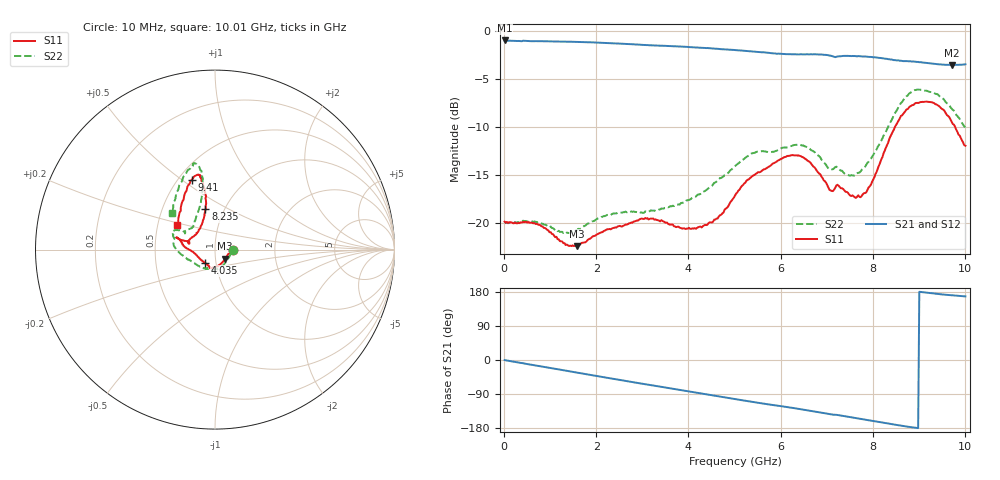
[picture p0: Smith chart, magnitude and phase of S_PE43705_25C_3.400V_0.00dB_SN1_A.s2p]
! Device ID: PE43705
! Serial: 1
! Insertion: A
! Impedance: 50 ohm
! Temp: 25C
! VDD: 3.400V
! Attenuation Step: 0.00dB
#  Hz  S  RI  R  50
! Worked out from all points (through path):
!   401 points, 10 MHz to 10.01 GHz, reference 50 ohm
!   highest |S21| = -0.98 dB at 10 MHz (marker M1); lowest = -3.5 dB at 9.71 GHz (marker M2)
!   group delay of S21, straight-line fit = 54.6 ps
!   lowest |S11| = -22.4 dB at 1.585 GHz (marker M3), VSWR 1.16, Z = 55.7 - j5.62 ohm
!   |S11| at or under -10 dB: start of sweep to 8.481 GHz; 9.787 GHz to end of sweep
!   |S22| runs from -21.1 to -6.1 dB; largest |S21 - S12| = 0.007
!   S11 on the Smith chart (normalised r, x): 10 MHz: 1.23, -0.00; 4.035 GHz: 0.88, -0.13; 8.235 GHz: 0.82, +0.39; 9.41 GHz: 0.58, +0.55; 10.01 GHz: 0.63, +0.18
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1e7  0.1015 -0.000899  0.8934 -0.00434  0.8937 -0.00403  0.1012 -0.000693
7.1e8  0.098 0.0132  0.8555 -0.2285  0.8556 -0.2284  0.1009 0.00697
1.585e9  0.0565 -0.0502  0.7331 -0.4824  0.7333 -0.4826  0.063 -0.0666
1.685e9  0.0506 -0.0603  0.7144 -0.5082  0.7143 -0.5085  0.0545 -0.0771
2.535e9  0.00155 -0.0959  0.5155 -0.6875  0.5163 -0.687  -0.0119 -0.1124
3.36e9  -0.0278 -0.099  0.2897 -0.7882  0.2903 -0.7875  -0.0524 -0.105
4.035e9  -0.0574 -0.0735  0.0935 -0.8192  0.0941 -0.8188  -0.1027 -0.0835
4.585e9  -0.0965 -0.0389  -0.0649 -0.8078  -0.0645 -0.8074  -0.1533 -0.0544
5.01e9  -0.1388 -0.003  -0.1801 -0.7753  -0.1796 -0.7753  -0.1966 -0.019
5.41e9  -0.1754 0.0211  -0.2793 -0.7305  -0.2787 -0.7312  -0.2298 0.0257
6.11e9  -0.2105 0.0663  -0.4201 -0.6309  -0.4161 -0.631  -0.2321 0.0839
6.685e9  -0.1922 0.055  -0.5318 -0.5375  -0.532 -0.5367  -0.2112 0.1099
7.085e9  -0.1422 0.0394  -0.5958 -0.4465  -0.5967 -0.4474  -0.1673 0.0913
7.26e9  -0.1478 0.0497  -0.6085 -0.418  -0.6066 -0.4192  -0.1569 0.1093
7.685e9  -0.1036 0.0929  -0.6671 -0.3216  -0.6666 -0.3216  -0.1189 0.1382
7.91e9  -0.0792 0.1309  -0.685 -0.2625  -0.6856 -0.2665  -0.1053 0.1799
8.235e9  -0.0538 0.2243  -0.6981 -0.1794  -0.6962 -0.1837  -0.0777 0.2744
8.36e9  -0.0502 0.2696  -0.6977 -0.147  -0.6961 -0.1499  -0.0711 0.3197
8.86e9  -0.0831 0.4028  -0.6937 -0.027  -0.6902 -0.0305  -0.102 0.4727
9.41e9  -0.1299 0.3893  -0.6688 0.0679  -0.6668 0.0675  -0.1515 0.4422
9.71e9  -0.174 0.2884  -0.6572 0.1073  -0.6555 0.1064  -0.2033 0.3379
1.001e10  -0.2116 0.1374  -0.6561 0.1413  -0.6586 0.1388  -0.2421 0.2013
